(* Logix 5000 Rung export; software revision 16.03 *)

MODULES
   Local : vendor None type None code None
   DPM : vendor None type None code None
END_MODULES

TYPE DDLM_SLAVE_DIAGNOSTIC_CONFIRM :
STRUCT
   Reserved1 : INT;
   Reserved2 : INT;
   Answer : SINT;
   Failure : SINT;
   Reserved3 : INT;
   DeviceAdr : SINT;
   DataArea : SINT;
   DataAdr : INT;
   DataIdx : SINT;
   DataCnt : SINT;
   DataType : SINT;
   Function : SINT;
   StationState_1 : SINT;
   StationState_2 : SINT;
   StationState_3 : SINT;
   MasterAddress : SINT;
   IdentNumber : INT;
   Reserved4 : INT;
   ExtDiag : SINT[100];
END_STRUCT
END_TYPE

TYPE DPM_DPV1_ALARM_INDICATION :   // DPV1 Alarm Indication
STRUCT
   AlarmIndication : BOOL;   // Indicates an alarm
   Reserved1 : BOOL;
   Reserved2 : BOOL;
   Reserved3 : BOOL;
   Reserved4 : BOOL;
   Reserved5 : BOOL;
   Reserved6 : BOOL;
   AlarmOverrun : BOOL;   // Overflow of the modules internal alarm buffer
   AlarmCnt : SINT;   // Alarm indication counter
   RemoteAddress : SINT;   // Address of Slave with Alarm
   Slot : SINT;   // Slot Number
   Sequence : SINT;   // Sequence Number
   AlarmType : SINT;   // Alarm Type
   AlarmSpec : SINT;   // Alarm Specification
   Reserved7 : SINT;
END_STRUCT
END_TYPE

TYPE DPM_INPUT_ARRAY :
STRUCT
   DevStaReg : DPM_DEV_STATUS_REGISTER;
   FwRev : DPM_FW_REVISION;
   GlobStateField : DPM_GLOBAL_STATE_FIELD;
   SlaveDiag : DPM_SLAVE_DIAG_DATA;
   AlarmInd : DPM_DPV1_ALARM_INDICATION;
   InputData : SINT[408];   // PROFIBUS Input data.
END_STRUCT
END_TYPE

TYPE DPM_GLOBAL_STATE_FIELD :   // PROFIBUS Master Global State Field
STRUCT
   Ctrl : BOOL;   // Control error
   Aclr : BOOL;   // Auto clear error
   Nexc : BOOL;   // Non exchange error
   Fat : BOOL;   // Fatal error
   Eve : BOOL;   // Event error
   NRdy : BOOL;   // Host not ready notification
   Tout : BOOL;   // Timeout
   Reserved1 : BOOL;   // Reserved
   DPM_State : SINT;   // Master main state
   Err_rem_adr : SINT;   // Faulty remote address
   Err_event : SINT;   // Error Number
   Bus_err_cnt : INT;   // Heavy bus error counter
   Time_out_cnt : INT;   // Number of rejected PROFIBUS Telegr.
   Reserved : SINT[8];   // Reserved
   Sl_cfg : BOOL[128];   // Slave Config
   Sl_state : BOOL[128];   // Slave State
   Sl_diag : BOOL[128];   // Slave Diag
END_STRUCT
END_TYPE

TYPE DDLM_SLAVE_DIAGNOSTIC_REQUEST :
STRUCT
   Reserved1 : INT;
   Reserved2 : INT;
   Reserved3 : INT;
   Command : SINT;
   Reserved4 : SINT;
   DeviceAdr : SINT;
   DataArea : SINT;
   DataAdr : INT;
   DataIdx : SINT;
   DataCnt : SINT;
   DataType : SINT;
   Function : SINT;
END_STRUCT
END_TYPE

TYPE DPM_OUTPUT_ARRAY :
STRUCT
   DevCmdReg : DPM_DEV_COMMAND_REGISTER;
   DiagReqAdr : DPM_SLAVE_DIAG_COMMAND;
   GlobCtrl : DPM_GLOBAL_CONTROL_COMMAND;
   Reserved : SINT[4];
   OutputData : SINT[480];   // PROFIBUS Output data.
END_STRUCT
END_TYPE

TYPE DPM_GLOBAL_CONTROL_COMMAND :   // Global Control Command
STRUCT
   SlaveAddress : SINT;   // Slave Address
   ControlCommand : SINT;   // Control Command to be send
   GroupSelect : SINT;   // Group Select
   Reserved1 : SINT;
END_STRUCT
END_TYPE

TYPE DPM_DEV_COMMAND_REGISTER :   // Device Command Register
STRUCT
   Reserved0 : BOOL;   // Reserved
   Reserved1 : BOOL;   // Reserved
   Reserved2 : BOOL;   // Reserved
   Reserved3 : BOOL;   // Reserved
   Reserved4 : BOOL;   // Reserved
   NRdy : BOOL;   // Application Not Ready
   Init : BOOL;   // Init ( Warm boot )
   Reset : BOOL;   // Reset ( Cold boot )
   HsReq0 : BOOL;   // Slave Diag Request
   HsReq1 : BOOL;   // Global Control Request
   HsReq2 : BOOL;   // Reserved
   HsReq3 : BOOL;   // Reserved
   HsReq4 : BOOL;   // Reserved
   HsReq5 : BOOL;   // Reserved
   HsReq6 : BOOL;   // Reserved
   HsReq7 : BOOL;   // Reserved
   Reserved5 : SINT;   // Reserved
   Reserved6 : SINT;   // Reserved
END_STRUCT
END_TYPE

TYPE MSAL1M_ALARM_RESPONSE :
STRUCT
   Reserved1 : INT;
   Reserved2 : INT;
   Reserved3 : INT;
   Command : SINT;
   Reserved4 : SINT;
   SlaveAdr : SINT;
   SlotNum : SINT;
   SeqNum : SINT;
   AlarmType : SINT;
   AlarmSpec : SINT;
   Reserved5 : SINT;
END_STRUCT
END_TYPE

TYPE DDLM_GLOBAL_CONTROL_REQUEST :
STRUCT
   Reserved1 : INT;
   Reserved2 : INT;
   Reserved3 : INT;
   Command : SINT;
   Reserved4 : SINT;
   DeviceAdr : SINT;
   ConrolCommand : SINT;
   GroupSelect : SINT;
END_STRUCT
END_TYPE

TYPE MSAC1_READ_REQUEST :   // DPV1 Read Request
STRUCT
   Reserved1 : INT;
   Reserved2 : INT;
   Reserved3 : INT;
   Command : SINT;
   Reserved4 : SINT;
   DeviceAdr : SINT;
   DataArea : SINT;
   DataAdr : INT;
   DataIdx : SINT;
   DataCnt : SINT;
   DataType : SINT;
   Function : SINT;
END_STRUCT
END_TYPE

TYPE MSAC1_READ_CONFIRM :   // DPV1 Read Confirmation
STRUCT
   Reserved1 : INT;
   Reserved2 : INT;
   Answer : SINT;
   Failure : SINT;
   Reserved3 : INT;
   DeciceAdr : SINT;
   DataArea : SINT;
   DataAdr : INT;
   DataIdx : SINT;
   DataCnt : SINT;
   DataType : SINT;
   Function : SINT;
   Data : SINT[240];
END_STRUCT
END_TYPE

TYPE MSAC1_WRITE_CONFIRM :   // DPV1 Write Confirmation
STRUCT
   Reserved1 : INT;
   Reserved2 : INT;
   Answer : SINT;
   Failure : SINT;
   Reserved3 : INT;
   DeciceAdr : SINT;
   DataArea : SINT;
   DataAdr : INT;
   DataIdx : SINT;
   DataCnt : SINT;
   DataType : SINT;
   Function : SINT;
   ErrorCode1 : SINT;
   ErrorCode2 : SINT;
END_STRUCT
END_TYPE

TYPE DPM_MODULEDEF :
STRUCT
   AlarmCnf : MSAL1M_ALARM_CONFIRM;
   AlarmIndCounter : SINT;
   AlarmReceiveCounter : INT;   // Alarm Counter
   AlarmResErr : BOOL;
   AlarmRsp : MSAL1M_ALARM_RESPONSE;
   DoDDLMGlblCtrl : BOOL;
   DoDDLMSetPrm : BOOL;
   DoDDLMSlaveDiag : BOOL;
   DoDPV1AlarmRsp : BOOL;
   DoDPV1ReadReq : BOOL;
   DoDPV1WriteReq : BOOL;
   DpmInputArray : DPM_INPUT_ARRAY;
   DpmOutputArray : DPM_OUTPUT_ARRAY;
   GlbCtrlCnf : DDLM_GLOBAL_CONTROL_CONFIRM;   // Global Control Confirmation
   GlbCtrlReq : DDLM_GLOBAL_CONTROL_REQUEST;   // Global Control Request
   MainInitDone : BOOL;
   ReadCnf : MSAC1_READ_CONFIRM;   // Read Confimation
   ReadReq : MSAC1_READ_REQUEST;   // Read Request
   SetPrmCnf : DDLM_SET_PARAMETER_CONFIRM;   // Set parameter confirmation
   SetPrmReq : DDLM_SET_PARAMETER_REQUEST;   // Set parameter request
   SlaveAddress : SINT;   // Slave address used by several CIP messages
   SlaveDiagCnf : DDLM_SLAVE_DIAGNOSTIC_CONFIRM;   // Slave Diag Confirmation
   SlaveDiagReq : DDLM_SLAVE_DIAGNOSTIC_REQUEST;   // Slave Diag Request
   WriteCnf : MSAC1_WRITE_CONFIRM;   // Slave Write Confirmation
   WriteReq : MSAC1_WRITE_REQUEST;   // Slave Write Request
END_STRUCT
END_TYPE

TYPE MSAL1M_ALARM_CONFIRM :
STRUCT
   Reserved1 : INT;
   Reserved2 : INT;
   Answer : SINT;
   Failure : SINT;
   Reserved3 : INT;
   SlaveAdr : SINT;
   SlotNum : SINT;
   SeqNum : SINT;
   AlarmType : SINT;
   AlarmSpec : SINT;
   Reserved4 : SINT;
END_STRUCT
END_TYPE

TYPE DPM_SLAVE_DIAG_COMMAND :   // Requested address for SlaveDiagnostics
STRUCT
   SlaveAddress : SINT;
   DiagMode : SINT;
   Reserved1 : SINT;
   Reserved2 : SINT;
END_STRUCT
END_TYPE

TYPE DPM_FW_REVISION :   // Firmware Major/Minor Revision
STRUCT
   FwMinor : SINT;   // Firmware Minor Revison
   FwMajor : SINT;   // Firmware Major Revison
   Reserved : INT;   // Reserved
END_STRUCT
END_TYPE

TYPE DPM_SLAVE_DIAG_DATA :   // Slave standard diagnostic data according to PROFIBUS norm.
STRUCT
   SlaveAddress : SINT;   // Slave address
   DiagFailure : SINT;   // Slave Diag Failure
   Sta1_StationNotExist : BOOL;   // No response
   Sta1_StationNotReady : BOOL;   // Station not ready
   Sta1_CfgFault : BOOL;   // Configuration faulty
   Sta1_ExtDiag : BOOL;   // Extended diagnostic
   Sta1_NotSupp : BOOL;   // Sync,Freeze not supported
   Sta1_InvalidResponse : BOOL;   // Response faulty
   Sta1_PrmFault : BOOL;   // Parameters faulty
   Sta1_MasterLock : BOOL;   // Locked by a master
   Sta2_PrmReq : BOOL;   // Request new parameter
   Sta2_StatDiag : BOOL;   // Static diagnostic
   Sta2_Slave : BOOL;   // Set to 1 by a slave
   Sta2_Watchdog : BOOL;   // Watchdog ON/OFF
   Sta2_FreezeMode : BOOL;   // Freeze mode active
   Sta2_SyncMode : BOOL;   // Sync mode active
   Sta2_Reserved : BOOL;   // Reserved
   Sta2_Deactivated : BOOL;   // Slave deactivated
   Sta3_Reserved0 : BOOL;   // Reserved
   Sta3_Reserved1 : BOOL;   // Reserved
   Sta3_Reserved2 : BOOL;   // Reserved
   Sta3_Reserved3 : BOOL;   // Reserved
   Sta3_Reserved4 : BOOL;   // Reserved
   Sta3_Reserved5 : BOOL;   // Reserved
   Sta3_Reserved6 : BOOL;   // Reserved
   Sta3_ExtDiagOverflow : BOOL;   // Extended diagnostic overflow
   MasterAddress : SINT;   // Corresponding master address
   IdentNumber : INT;   // PROFIBUS Ident number
END_STRUCT
END_TYPE

TYPE DPM_DEV_STATUS_REGISTER :   // Device Status Register
STRUCT
   Reserved0 : BOOL;
   Reserved1 : BOOL;
   Reserved2 : BOOL;
   Reserved3 : BOOL;
   Reserved4 : BOOL;
   Com : BOOL;   // Communication
   Run : BOOL;   // Running
   Rdy : BOOL;   // Ready
   HsAck0 : BOOL;   // Slave Diag Acknowledge
   HsAck1 : BOOL;   // Global Control Acknowledge
   HsAck2 : BOOL;
   HsAck3 : BOOL;
   HsAck4 : BOOL;
   HsAck5 : BOOL;
   HsAck6 : BOOL;
   HsAck7 : BOOL;
   Reserved5 : SINT;
   Reserved6 : SINT;
END_STRUCT
END_TYPE

TYPE DDLM_GLOBAL_CONTROL_CONFIRM :
STRUCT
   Reserved1 : INT;
   Reserved2 : INT;
   Answer : SINT;
   Failure : SINT;
   Reserved3 : INT;
   DeviceAdr : SINT;
END_STRUCT
END_TYPE

TYPE DDLM_SET_PARAMETER_REQUEST :
STRUCT
   Reserved1 : INT;
   Reserved2 : INT;
   Reserved3 : INT;
   Command : SINT;
   Reserved4 : SINT;
   UsrPrm : SINT[234];
END_STRUCT
END_TYPE

TYPE DDLM_SET_PARAMETER_CONFIRM :
STRUCT
   Reserved1 : INT;
   Reserved2 : INT;
   Answer : SINT;
   Failure : SINT;
   Reserved3 : INT;
   DeviceAdr : SINT;
END_STRUCT
END_TYPE

TYPE MSAC1_WRITE_REQUEST :   // DPV1 Write Request
STRUCT
   Reserved1 : INT;
   Reserved2 : INT;
   Reserved3 : INT;
   Command : SINT;
   Reserved4 : SINT;
   DeviceAdr : SINT;
   DataArea : SINT;
   DataAdr : INT;
   DataIdx : SINT;
   DataCnt : SINT;
   DataType : SINT;
   Function : SINT;
   data : SINT[240];
END_STRUCT
END_TYPE

ADD_ON_INSTRUCTION AOIPS69DPM   (* revision 1.1, vendor Prosoft Technology Inc *)
// Add-On instruction for the PS69-DPM module
// Revision note:
// Added viewing capability for the Add_On Instruction
VAR_IN_OUT
   Connection_Input : INT[248]; {required}
   Connection_Output : INT[248]; {required}
   PS69DPM : DPM_MODULEDEF; {required}
   AlarmRspMsg : MESSAGE; {required}
   GlbCtrlMsg : MESSAGE; {required}
   ReadReqMsg : MESSAGE; {required}
   SetPrmReqMsg : MESSAGE; {required}
   SlaveDiagMsg : MESSAGE; {required}
   WriteReqMsg : MESSAGE; {required}
END_VAR

ROUTINE Logic   (* ladder *)
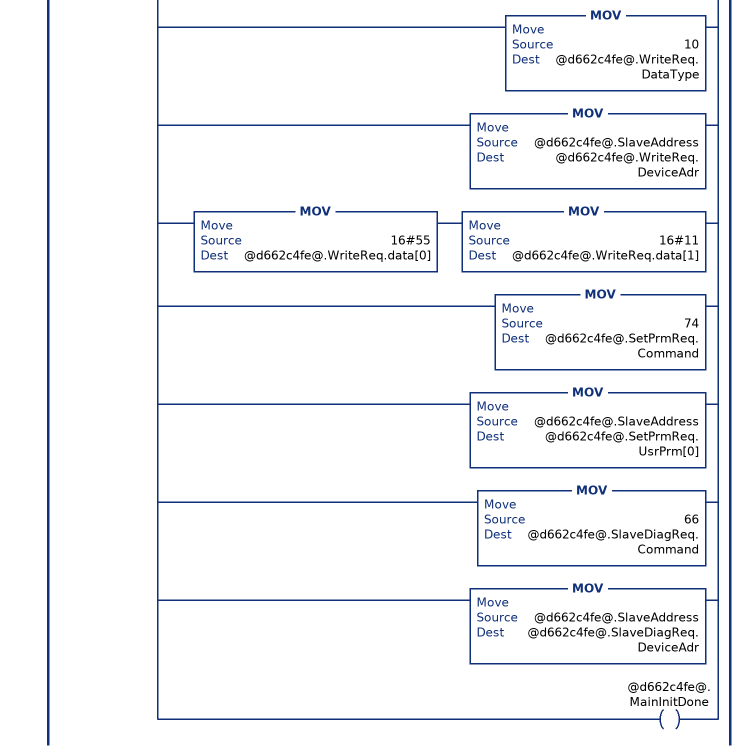
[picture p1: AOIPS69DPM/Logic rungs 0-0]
   // Vendor/Address/Phone/Product (revs) /Description/ACDname (date)
   // Prosoft Technology Inc
   // 1675 Chester Avenue, Fourth Floor
   // Bakersfield, CA 93301
   // USA
   // Phone: 1-661-7165100
   // PS69-DPM
   // PROFIBUS-DP Master Module
   // PS69_DPM_messaging_L32E.ACD (Rev1.0) (07/28/05)
   // Although this program has been developed with great care and intensively tested,
   // Prosoft Technology Inc cannot guarantee the suitability of this program
   // for any purpose not confirmed by us in writing.
   // We reserve the right to modify our products and their specifications at any time in as far as this contributes to technical progress.
   // The version of the manual supplied with the program applies.
   // Guarantee claims shall be limited to the right to require rectification. Liability for any damages which may have arisen from the use of this program or its documentation shall be limited to cases of intent.
   // This program is a basic example RSLogix5000 project used for sending PROFIBUS messages to the communication module "PS69-DPM". This project provides an example for every supported PROFIBUS message by the module.
   // For detailed information about the these messages (functionality, parameters, error codes etc. ) refer to the module User Manual.
   // Rung 0 calls all init routines for one time, to initialize the PROFIBUS commands.
   0: XIO(@d662c4fe@.MainInitDone)[MOV(18,@d662c4fe@.AlarmRsp.Command) ,MOV(70,@d662c4fe@.GlbCtrlReq.Command) ,MOV(@d662c4fe@.SlaveAddress,@d662c4fe@.GlbCtrlReq.DeviceAdr) ,MOV(17,@d662c4fe@.ReadReq.Command) ,MOV(1,@d662c4fe@.ReadReq.Function) ,MOV(@d662c4fe@.SlaveAddress,@d662c4fe@.ReadReq.DeviceAdr) ,MOV(10,@d662c4fe@.ReadReq.DataType) ,MOV(17,@d662c4fe@.WriteReq.Command) ,MOV(2,@d662c4fe@.WriteReq.Function) ,MOV(10,@d662c4fe@.WriteReq.DataType) ,MOV(@d662c4fe@.SlaveAddress,@d662c4fe@.WriteReq.DeviceAdr) ,MOV(16#55,@d662c4fe@.WriteReq.data[0]) MOV(16#11,@d662c4fe@.WriteReq.data[1]) ,MOV(74,@d662c4fe@.SetPrmReq.Command) ,MOV(@d662c4fe@.SlaveAddress,@d662c4fe@.SetPrmReq.UsrPrm[0]) ,MOV(66,@d662c4fe@.SlaveDiagReq.Command) ,MOV(@d662c4fe@.SlaveAddress,@d662c4fe@.SlaveDiagReq.DeviceAdr) ,OTE(@d662c4fe@.MainInitDone) ];
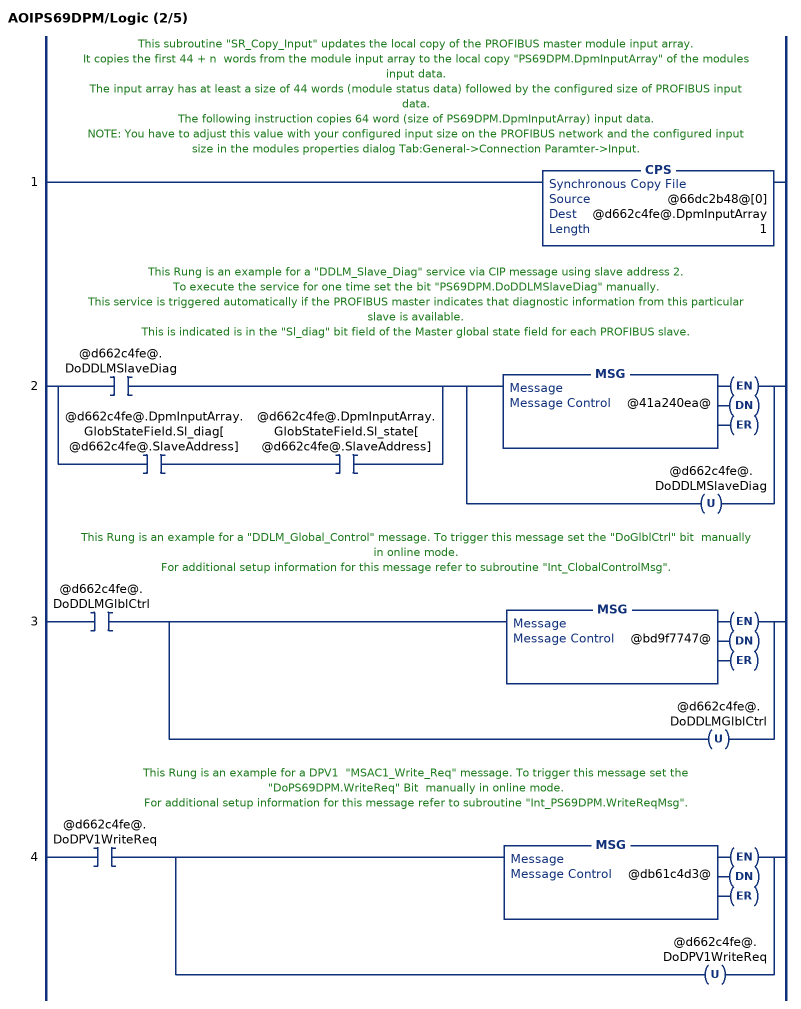
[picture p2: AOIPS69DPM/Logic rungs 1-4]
   // This subroutine "SR_Copy_Input" updates the local copy of the PROFIBUS master module input array.
   // It copies the first 44 + n  words from the module input array to the local copy "PS69DPM.DpmInputArray" of the modules input data.
   // The input array has at least a size of 44 words (module status data) followed by the configured size of PROFIBUS input data.
   // The following instruction copies 64 word (size of PS69DPM.DpmInputArray) input data.
   // NOTE: You have to adjust this value with your configured input size on the PROFIBUS network and the configured input size in the modules properties dialog Tab:General->Connection Paramter->Input.
   1: CPS(@66dc2b48@[0],@d662c4fe@.DpmInputArray,1);
   // This Rung is an example for a "DDLM_Slave_Diag" service via CIP message using slave address 2.
   // To execute the service for one time set the bit "PS69DPM.DoDDLMSlaveDiag" manually.
   // This service is triggered automatically if the PROFIBUS master indicates that diagnostic information from this particular slave is available.
   // This is indicated is in the "Sl_diag" bit field of the Master global state field for each PROFIBUS slave.
   2: [XIC(@d662c4fe@.DoDDLMSlaveDiag) ,XIC(@d662c4fe@.DpmInputArray.GlobStateField.Sl_diag[@d662c4fe@.SlaveAddress]) XIC(@d662c4fe@.DpmInputArray.GlobStateField.Sl_state[@d662c4fe@.SlaveAddress]) ][MSG(@41a240ea@) ,OTU(@d662c4fe@.DoDDLMSlaveDiag) ];
   // This Rung is an example for a "DDLM_Global_Control" message. To trigger this message set the "DoGlblCtrl" bit  manually in online mode.
   // For additional setup information for this message refer to subroutine "Int_ClobalControlMsg".
   3: XIC(@d662c4fe@.DoDDLMGlblCtrl)[MSG(@bd9f7747@) ,OTU(@d662c4fe@.DoDDLMGlblCtrl) ];
   // This Rung is an example for a DPV1  "MSAC1_Write_Req" message. To trigger this message set the "DoPS69DPM.WriteReq" Bit  manually in online mode.
   // For additional setup information for this message refer to subroutine "Int_PS69DPM.WriteReqMsg".
   4: XIC(@d662c4fe@.DoDPV1WriteReq)[MSG(@db61c4d3@) ,OTU(@d662c4fe@.DoDPV1WriteReq) ];
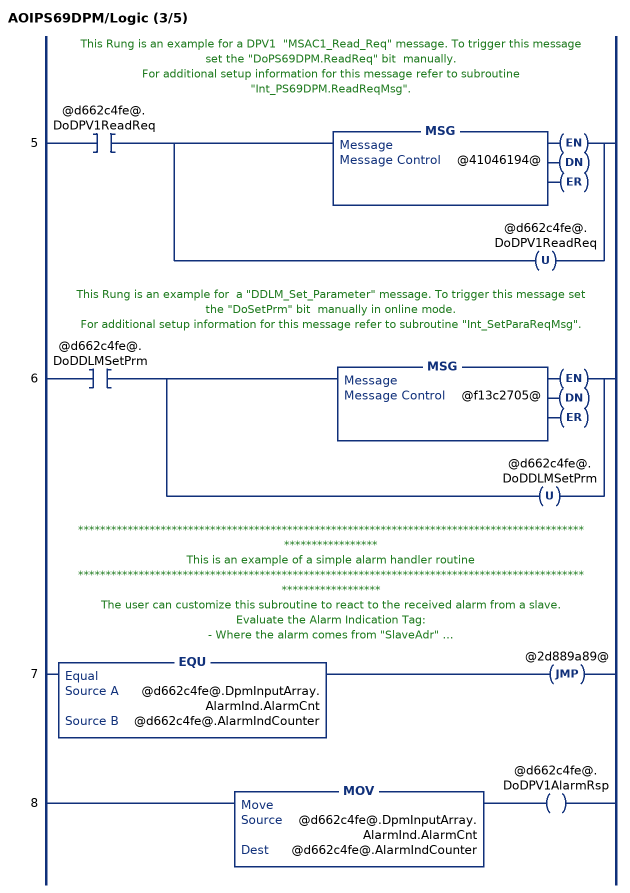
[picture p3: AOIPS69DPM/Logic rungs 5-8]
   // This Rung is an example for a DPV1  "MSAC1_Read_Req" message. To trigger this message set the "DoPS69DPM.ReadReq" bit  manually.
   // For additional setup information for this message refer to subroutine "Int_PS69DPM.ReadReqMsg".
   5: XIC(@d662c4fe@.DoDPV1ReadReq)[MSG(@41046194@) ,OTU(@d662c4fe@.DoDPV1ReadReq) ];
   // This Rung is an example for  a "DDLM_Set_Parameter" message. To trigger this message set the "DoSetPrm" bit  manually in online mode.
   // For additional setup information for this message refer to subroutine "Int_SetParaReqMsg".
   6: XIC(@d662c4fe@.DoDDLMSetPrm)[MSG(@f13c2705@) ,OTU(@d662c4fe@.DoDDLMSetPrm) ];
   // *************************************************************************************************************
   // This is an example of a simple alarm handler routine
   // **************************************************************************************************************
   // The user can customize this subroutine to react to the received alarm from a slave.
   // Evaluate the Alarm Indication Tag:
   //  - Where the alarm comes from "SlaveAdr" ?
   // -  What kind of alarm is it  "AlarmType" ?
   // ect. ....
   7: EQU(@d662c4fe@.DpmInputArray.AlarmInd.AlarmCnt,@d662c4fe@.AlarmIndCounter)JMP(@2d889a89@);
   8: MOV(@d662c4fe@.DpmInputArray.AlarmInd.AlarmCnt,@d662c4fe@.AlarmIndCounter)OTE(@d662c4fe@.DoDPV1AlarmRsp);
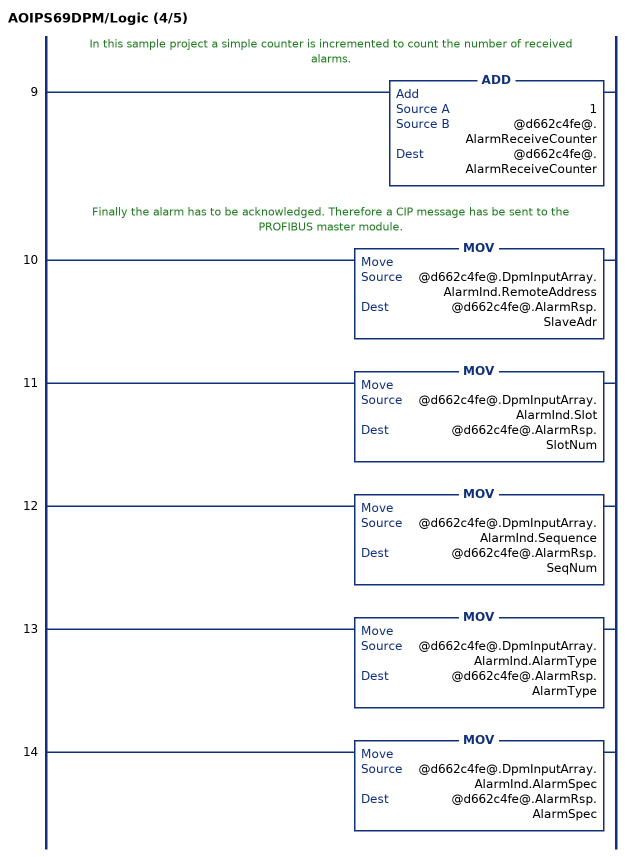
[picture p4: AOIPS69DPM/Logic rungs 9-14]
   // In this sample project a simple counter is incremented to count the number of received alarms.
   9: ADD(1,@d662c4fe@.AlarmReceiveCounter,@d662c4fe@.AlarmReceiveCounter);
   // Finally the alarm has to be acknowledged. Therefore a CIP message has be sent to the PROFIBUS master module.
   10: MOV(@d662c4fe@.DpmInputArray.AlarmInd.RemoteAddress,@d662c4fe@.AlarmRsp.SlaveAdr);
   11: MOV(@d662c4fe@.DpmInputArray.AlarmInd.Slot,@d662c4fe@.AlarmRsp.SlotNum);
   12: MOV(@d662c4fe@.DpmInputArray.AlarmInd.Sequence,@d662c4fe@.AlarmRsp.SeqNum);
   13: MOV(@d662c4fe@.DpmInputArray.AlarmInd.AlarmType,@d662c4fe@.AlarmRsp.AlarmType);
   14: MOV(@d662c4fe@.DpmInputArray.AlarmInd.AlarmSpec,@d662c4fe@.AlarmRsp.AlarmSpec);
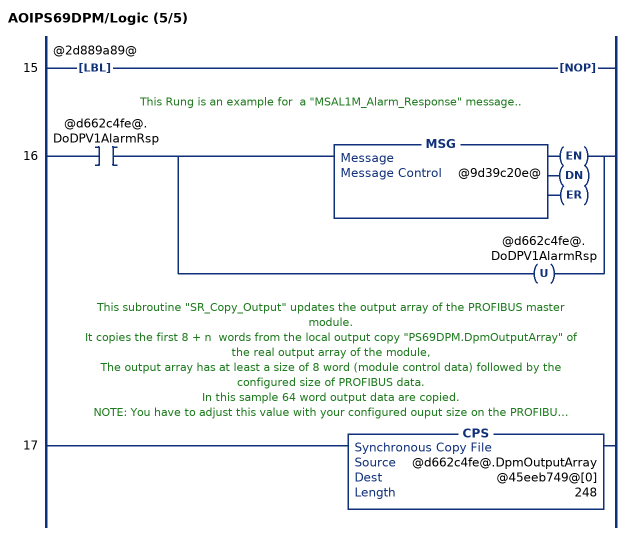
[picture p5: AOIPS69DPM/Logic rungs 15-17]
   15: LBL(@2d889a89@)NOP();
   // This Rung is an example for  a "MSAL1M_Alarm_Response" message..
   16: XIC(@d662c4fe@.DoDPV1AlarmRsp)[MSG(@9d39c20e@) ,OTU(@d662c4fe@.DoDPV1AlarmRsp) ];
   // This subroutine "SR_Copy_Output" updates the output array of the PROFIBUS master module.
   // It copies the first 8 + n  words from the local output copy "PS69DPM.DpmOutputArray" of the real output array of the module,
   // The output array has at least a size of 8 word (module control data) followed by the configured size of PROFIBUS data.
   // In this sample 64 word output data are copied.
   // NOTE: You have to adjust this value with your configured ouput size on the PROFIBUS network and the configured output size in the modules properties dialog Tab:General->Connection Paramter->Output.
   17: CPS(@d662c4fe@.DpmOutputArray,@45eeb749@[0],248);
END_ROUTINE
END_ADD_ON_INSTRUCTION

VAR_GLOBAL   (* controller tags *)
   Local:1:I : AB:1769_MODULE_INT_500Bytes:I:0;
   PS69DPM : DPM_MODULEDEF;
   SlaveDiagMsg : MESSAGE;   // Slave Diag Message
        .EN   // Slave Diag Message
        MessageParameters(MessageType := CIP Generic, RequestedLength := 16, ConnectedFlag := 2, ConnectionPath := DPM, ServiceCode := 16#0064, ObjectType := 16#0065, TargetObject := 1, LocalElement := PS69DPM.SlaveDiagReq, DestinationTag := PS69DPM.SlaveDiagCnf)
   WriteReqMsg : MESSAGE;   // Slave Write Request Message
        .EN   // Slave Write Request Message
        MessageParameters(MessageType := CIP Generic, RequestedLength := 18, ConnectedFlag := 2, ConnectionPath := DPM, ServiceCode := 16#0064, ObjectType := 16#0065, TargetObject := 1, LocalElement := PS69DPM.WriteReq, DestinationTag := PS69DPM.WriteCnf)
   AlarmRspMsg : MESSAGE;   // Alarm Response Message
        MessageParameters(MessageType := CIP Generic, RequestedLength := 14, ConnectedFlag := 2, ConnectionPath := DPM, ServiceCode := 16#0064, ObjectType := 16#0065, TargetObject := 1, LocalElement := PS69DPM.AlarmRsp, DestinationTag := PS69DPM.AlarmCnf)
   GlbCtrlMsg : MESSAGE;   // Global Control Message
        MessageParameters(MessageType := CIP Generic, RequestedLength := 11, ConnectedFlag := 2, ConnectionPath := DPM, ServiceCode := 16#0064, ObjectType := 16#0065, TargetObject := 1, LocalElement := PS69DPM.GlbCtrlReq, DestinationTag := PS69DPM.GlbCtrlCnf)
   SetPrmReqMsg : MESSAGE;
        MessageParameters(MessageType := CIP Generic, RequestedLength := 10, ConnectedFlag := 2, ConnectionPath := DPM, ServiceCode := 16#0064, ObjectType := 16#0065, TargetObject := 1, LocalElement := PS69DPM.SetPrmReq, DestinationTag := PS69DPM.SetPrmCnf)
   AOIPS69DPM : AOIPS69DPM;
   Local:1:O : AB:1769_MODULE_INT_496Bytes:O:0;
   ReadReqMsg : MESSAGE;   // Slave Read Request Message
        .EN   // Slave Read Request Message
        MessageParameters(MessageType := CIP Generic, RequestedLength := 16, ConnectedFlag := 2, ConnectionPath := DPM, ServiceCode := 16#0064, ObjectType := 16#0065, TargetObject := 1, LocalElement := PS69DPM.ReadReq, DestinationTag := PS69DPM.ReadCnf)
END_VAR

PROGRAM MainProgram

ROUTINE MainRoutine   (* ladder *)
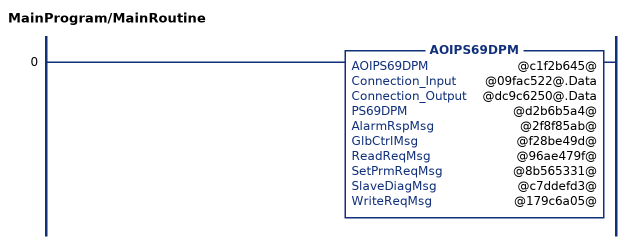
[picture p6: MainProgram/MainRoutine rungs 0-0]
   0: AOIPS69DPM(@c1f2b645@,@09fac522@.Data,@dc9c6250@.Data,@d2b6b5a4@,@2f8f85ab@,@f28be49d@,@96ae479f@,@8b565331@,@c7ddefd3@,@179c6a05@);
END_ROUTINE
END_PROGRAM
